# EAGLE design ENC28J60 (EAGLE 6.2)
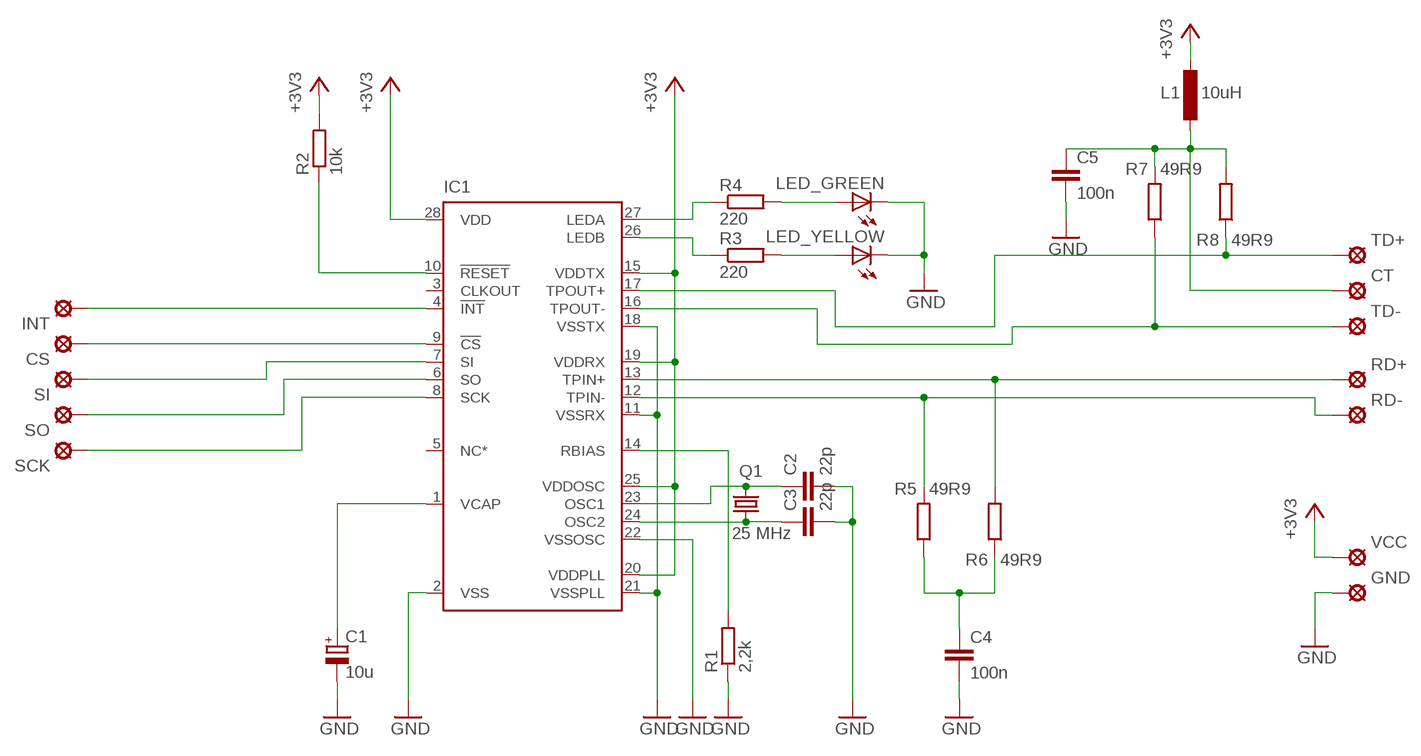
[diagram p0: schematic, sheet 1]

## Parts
C1  10u  CPOL-EUE/7260-38R  [E/7260-38R]
C2  22p  C-EUC1206  [C1206]
C3  22p  C-EUC1206  [C1206]
C4  100n  C-EUC1206  [C1206]
C5  100n  C-EUC1206  [C1206]
CS  SE14  [SE14]
CT  SE14  [SE14]
GND  SE14  [SE14]
IC1  ENC28J60SO  [SO28W]
INT  SE14  [SE14]
L1  10uH  L-EUL1812  [L1812]
LED_GREEN  LEDKA-3528ASYC  [KA-3528ASYC]
LED_YELLOW  LEDKA-3528ASYC  [KA-3528ASYC]
Q1  25 MHz  CRYSTALHC49U-V  [HC49U-V]
R1  2,2k  R-EU_R1206  [R1206]
R2  10k  R-EU_M1206  [M1206]
R3  220  R-EU_M1206  [M1206]
R4  220  R-EU_M1206  [M1206]
R5  49R9  R-EU_M1206  [M1206]
R6  49R9  R-EU_M1206  [M1206]
R7  49R9  R-EU_M1206  [M1206]
R8  49R9  R-EU_M1206  [M1206]
RD+  SE14  [SE14]
RD-  SE14  [SE14]
SCK  SE14  [SE14]
SI  SE14  [SE14]
SO  SE14  [SE14]
TD+  SE14  [SE14]
TD-  SE14  [SE14]
VCC  SE14  [SE14]

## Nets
+3V3: IC1.15(VDDTX) IC1.19(VDDRX) IC1.20(VDDPLL) IC1.25(VDDOSC) IC1.28(VDD) L1.1 R2.2 VCC.MP
/INT: IC1.4(!INT) INT.MP
GND: C1.- C2.2 C3.2 C4.2 C5.2 GND.MP IC1.2(VSS) IC1.11(VSSRX) IC1.18(VSSTX) IC1.21(VSSPLL) IC1.22(VSSOSC) LED_GREEN.C LED_YELLOW.C R1.1
N$1: IC1.14(RBIAS) R1.2
N$2: C1.+ IC1.1(VCAP)
N$3: C3.1 IC1.24(OSC2) Q1.1
N$4: C2.1 IC1.23(OSC1) Q1.2
N$5: IC1.17(TPOUT+) R8.1 TD+.MP
N$6: IC1.16(TPOUT-) R7.1 TD-.MP
N$7: IC1.12(TPIN-) R5.2 RD-.MP
N$8: IC1.13(TPIN+) R6.2 RD+.MP
N$9: IC1.10(!RESET) R2.1
N$10: C4.1 R5.1 R6.1
N$11: C5.1 CT.MP L1.2 R7.2 R8.2
N$12: IC1.27(LEDA) R4.1
N$13: IC1.26(LEDB) R3.1
N$14: LED_GREEN.A R4.2
N$15: LED_YELLOW.A R3.2
N$18: CS.MP IC1.9(!CS)
N$19: IC1.7(SI) SI.MP
N$20: IC1.6(SO) SO.MP
N$21: IC1.8(SCK) SCK.MP
Unconnected: IC1.3(CLKOUT) IC1.5(NC*)

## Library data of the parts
C1 = resistor:CPOL-EU: POLARIZED CAPACITOR, European symbol
C2-C5 = rcl:C-EU: CAPACITOR, European symbol
CS CT GND INT RD+ RD- SCK SI SO TD+ TD- VCC = solpad:SE14: SOLDER PAD
IC1 = ENC28J60:ENC28J60: Stand-Alone Ethernet Controller with SPI Interface Source: http://ww1.microchip.com/downloads/en/DeviceDoc/39662c.pdf
L1 = rcl:L-EU: INDUCTOR, European symbol
LED_GREEN LED_YELLOW = led:LED: LED
Q1 = crystal:CRYSTAL: CRYSTAL; OC_FARNELL: 1666969; OC_NEWARK: unknown
R1-R8 = rcl:R-EU_: RESISTOR, European symbol

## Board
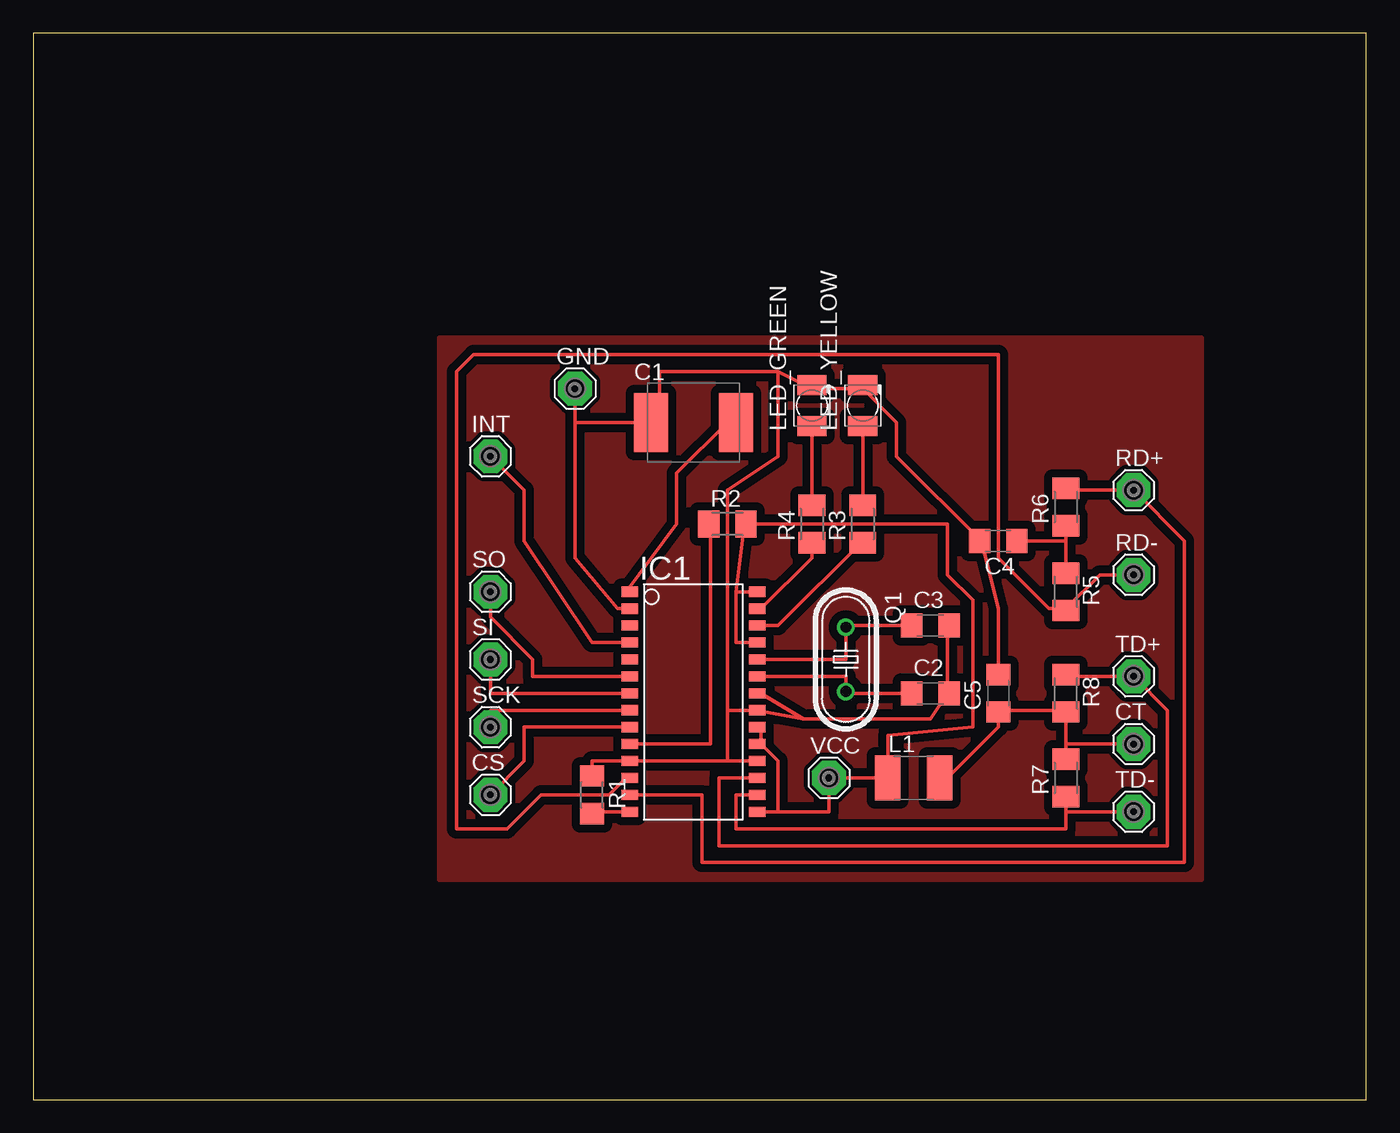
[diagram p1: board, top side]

Size 100 x 80 mm. Coordinates in mm from the lower left corner, seen from the top.
Outline: 0,0 100,0 100,80 0,80 0,0
Copper layers (1*16): Top 0.035mm / dielectric 1.5mm / Bottom 0.035mm
Design rules: minimum track width 10mil, minimum drill 24mil, track to track 8mil, track to pad 8mil, pad to pad 8mil, via to via 8mil, smd to smd 8mil, copper to edge 40mil, drill to drill 8mil, minimum pad ring 10mil, minimum via ring 8mil, stop-mask expansion 4mil, vias tented up to drill 0mil, thermal gap 10mil

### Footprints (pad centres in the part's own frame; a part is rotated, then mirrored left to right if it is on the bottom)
E/7260-38R = smd 2.55 x 4.4: + 3.175,0; - -3.175,0
C1206 = smd 1.6 x 1.8: 1 -1.4,0; 2 1.4,0
SE14 = drill 1.397 pad 2.54 octagon: MP 0,0
SO28W = smd 0.762 x 1.27: 1 -7.62,-4.78; 2 -6.35,-4.78; 3 -5.08,-4.78; 4 -3.81,-4.78; 5 -2.54,-4.78; 6 -1.27,-4.78; 7 0,-4.78; 8 1.27,-4.78; 9 2.54,-4.78; 10 3.81,-4.78; 11 5.08,-4.78; 12 6.35,-4.78; 13 7.62,-4.78; 14 8.89,-4.78; 15 8.89,4.78; 16 7.62,4.78; 17 6.35,4.78; 18 5.08,4.78; 19 3.81,4.78; 20 2.54,4.78; 21 1.27,4.78; 22 0,4.78; 23 -1.27,4.78; 24 -2.54,4.78; 25 -3.81,4.78; 26 -5.08,4.78; 27 -6.35,4.78; 28 -7.62,4.78
L1812 = smd 1.9 x 3.4: 1 -1.95,0; 2 1.95,0
KA-3528ASYC = smd 1.5 x 2.2: A -1.55,0; C 1.55,0
HC49U-V = drill 0.813: 1 -2.413,0; 2 2.413,0
R1206 = smd 1.6 x 1.803: 1 -1.422,0; 2 1.422,0
M1206 = smd 1.6 x 2: 1 -1.4,0; 2 1.4,0

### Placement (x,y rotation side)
C1  49.53,50.8 0 top
C2  67.31,30.48 0 top
C3  67.31,35.56 0 top
C4  72.39,41.91 180 top
C5  72.39,30.48 90 top
CS  34.29,22.86 0 top
CT  82.55,26.67 0 top
GND  40.64,53.34 0 top
IC1  49.53,30.48 270 top
INT  34.29,48.26 0 top
L1  66.04,24.13 0 top
LED_GREEN  58.42,52.07 90 top
LED_YELLOW  62.23,52.07 90 top
Q1  60.96,33.02 270 top
R1  41.91,22.86 270 top
R2  52.07,43.18 0 top
R3  62.23,43.18 90 top
R4  58.42,43.18 90 top
R5  77.47,38.1 270 top
R6  77.47,44.45 90 top
R7  77.47,24.13 90 top
R8  77.47,30.48 270 top
RD+  82.55,45.72 0 top
RD-  82.55,39.37 0 top
SCK  34.29,27.94 0 top
SI  34.29,33.02 0 top
SO  34.29,38.1 0 top
TD+  82.55,31.75 0 top
TD-  82.55,21.59 0 top
VCC  59.69,24.13 0 top

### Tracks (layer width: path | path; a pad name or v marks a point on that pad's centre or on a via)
+3V3
  Top 0.254: 52.7,38.1 53.34,43.18 R2.2 68.58,43.18 68.58,39.37 70.48,37.47 70.48,27.94 64.14,27.3 L1.1 VCC.MP 59.69,21.59 55.88,21.59 | 52.7,38.1 52.7,34.29 IC1.25 54.61,34.29 | 52.7,38.1 IC1.28 54.61,38.1 | 54.61,26.67 54.61,27.94 IC1.20 | 55.88,21.59 IC1.15 | 54.61,26.67 55.88,25.4 55.88,21.59 | 54.61,26.67 IC1.19
/INT
  Top 0.254: INT.MP 36.83,45.72 36.83,41.91 41.91,34.29 IC1.4
GND
  Top 0.254: 68.58,30.48 68.58,35.56 C3.2 | 57.78,28.57 54.61,30.48 IC1.22 | 41.91,24.13 R1.1 41.91,25.4 IC1.11 52.07,25.4 | 52.07,25.4 IC1.18 54.61,25.4 | 52.07,29.21 IC1.21 57.78,28.57 | 52.07,25.4 52.07,29.21 | 68.58,30.48 67.31,28.57 57.78,28.57 | 68.58,30.48 C2.2 | GND.MP 40.64,50.8 | 40.64,50.8 40.64,40.64 43.81,36.83 IC1.2 | 71.12,41.91 72.39,36.83 C5.2 72.39,31.75 | 62.23,53.34 58.42,53.34 | 55.88,54.61 46.99,54.61 46.99,50.8 C1.- 40.64,50.8 | 55.88,54.61 58.42,53.34 | 58.42,53.34 LED_GREEN.C | 71.12,41.91 64.77,48.26 64.77,50.8 62.23,53.34 | 71.12,41.91 C4.2 | 62.23,53.34 LED_YELLOW.C | 52.07,29.21 52.07,45.72 55.88,48.26 55.88,54.61
N$1
  Top 0.254: IC1.14 41.91,21.59 R1.2
N$2
  Top 0.254: IC1.1 44.45,38.1 48.26,43.18 48.26,46.99 52.07,50.8 C1.+
N$3
  Top 0.254: IC1.24 60.96,33.02 Q1.1 60.96,35.56 C3.1 66.04,35.56
N$4
  Top 0.254: IC1.23 60.96,31.75 Q1.2 60.96,30.48 C2.1 66.04,30.48
N$5
  Top 0.254: 54.61,24.13 IC1.17 51.44,24.13 51.44,19.05 85.09,19.05 85.09,29.21 TD+.MP 77.47,31.75 R8.1
N$6
  Top 0.254: 77.47,21.59 R7.1 77.47,22.86 | 77.47,21.59 77.47,20.32 52.7,20.32 52.7,22.86 IC1.16 54.61,22.86 | 77.47,21.59 TD-.MP
N$7
  Top 0.254: 77.47,36.83 76.2,36.83 72.39,40.64 72.39,55.88 33.02,55.88 31.75,54.61 31.75,20.32 35.56,20.32 38.1,22.86 43.18,22.86 44.45,24.13 IC1.12 | RD-.MP 80.01,39.37 77.47,36.83 | 77.47,36.83 R5.2
N$8
  Top 0.254: 44.45,22.86 IC1.13 50.16,22.86 50.16,17.78 86.36,17.78 86.36,41.91 RD+.MP 77.47,45.72 R6.2
N$9
  Top 0.254: 44.45,26.67 IC1.10 50.8,26.67 50.8,43.18 R2.1
N$10
  Top 0.254: 77.47,41.91 C4.1 73.66,41.91 | 77.47,41.91 R6.1 77.47,43.18 | 77.47,41.91 R5.1 77.47,39.37
N$11
  Top 0.254: 77.47,26.67 R8.2 77.47,29.21 72.39,29.21 C5.1 72.39,27.94 68.58,24.13 L1.2 | 77.47,26.67 R7.2 77.47,25.4 | 77.47,26.67 CT.MP
N$12
  Top 0.254: IC1.27 54.61,36.83 58.42,40.64 R4.1 58.42,41.91
N$13
  Top 0.254: IC1.26 55.88,35.56 62.23,41.91 R3.1
N$14
  Top 0.254: 58.42,44.45 R4.2 LED_GREEN.A 58.42,50.8
N$15
  Top 0.254: 62.23,44.45 R3.2 LED_YELLOW.A 62.23,50.8
N$18
  Top 0.254: IC1.9 36.83,27.94 36.83,25.4 CS.MP
N$19
  Top 0.254: IC1.7 34.29,30.48 SI.MP
N$20
  Top 0.254: IC1.6 37.47,31.75 37.47,33.02 34.29,36.2 SO.MP
N$21
  Top 0.254: IC1.8 34.29,29.21 SCK.MP
N$23
  pour Top (isolate 0.61): 87.63,16.51 30.48,16.51 30.48,57.15 87.63,57.15 87.63,55.88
